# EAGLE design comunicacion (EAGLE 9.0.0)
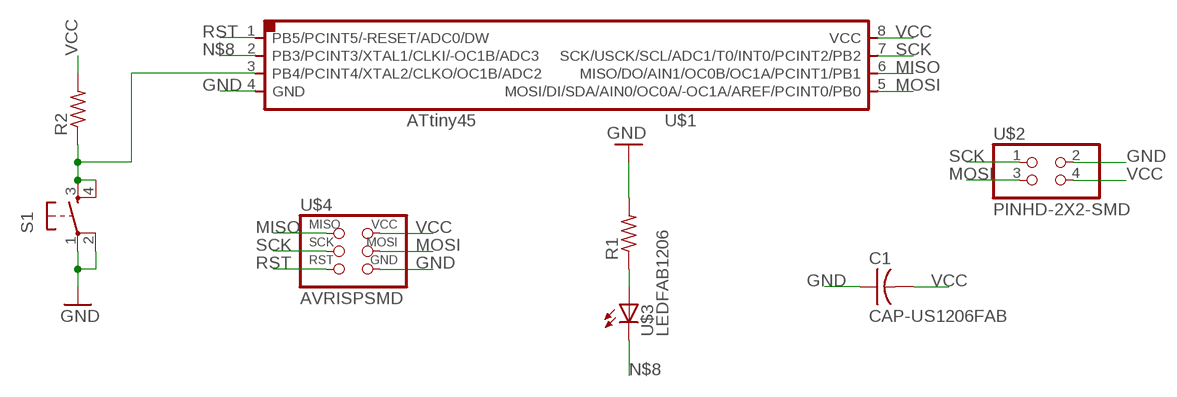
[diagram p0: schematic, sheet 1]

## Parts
C1  CAP-US1206FAB  [C1206FAB]
R1  RES-US1206FAB  [R1206FAB]
R2  RES-US1206FAB  [R1206FAB]
S1  6MM_SWITCH6MM_SWITCH  [6MM_SWITCH]
U$1  ATTINY45SI  [SOIC8]
U$2  PINHD-2X2-SMD  [2X02SMD]
U$3  LEDFAB1206  [LED1206FAB]
U$4  AVRISPSMD  [2X03SMD]

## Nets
GND: C1.1 R1.2 S1.1(P) S1.2(P1) U$1.4(GND) U$2.2 U$4.6(GND)
MISO: U$1.6(MISO/DO/AIN1/OC0B/OC1A/PCINT1/PB1) U$4.1(MISO)
MOSI: U$1.5(MOSI/DI/SDA/AIN0/OC0A/-OC1A/AREF/PCINT0/PB0) U$2.3 U$4.4(MOSI)
N$2: R2.1 S1.3(S) S1.4(S1) U$1.3(PB4/PCINT4/XTAL2/CLKO/OC1B/ADC2)
N$7: R1.1 U$3.1(A)
N$8: U$1.2(PB3/PCINT3/XTAL1/CLKI/-OC1B/ADC3) U$3.2(C)
RST: U$1.1(PB5/PCINT5/-RESET/ADC0/DW) U$4.5(RST)
SCK: U$1.7(SCK/USCK/SCL/ADC1/T0/INT0/PCINT2/PB2) U$2.1 U$4.3(SCK)
VCC: C1.2 R2.2 U$1.8(VCC) U$2.4 U$4.2(VCC)

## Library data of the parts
C1 = fab:CAP-US
R1 R2 = fab:RES-US: Resistor (US Symbol)
S1 = fab:6MM_SWITCH: OMRON SWITCH
U$1 = fab:ATTINY45
U$2 = fab:PINHD-2X2-SMD
U$3 = fab:LED: LED
U$4 = fab:AVRISP

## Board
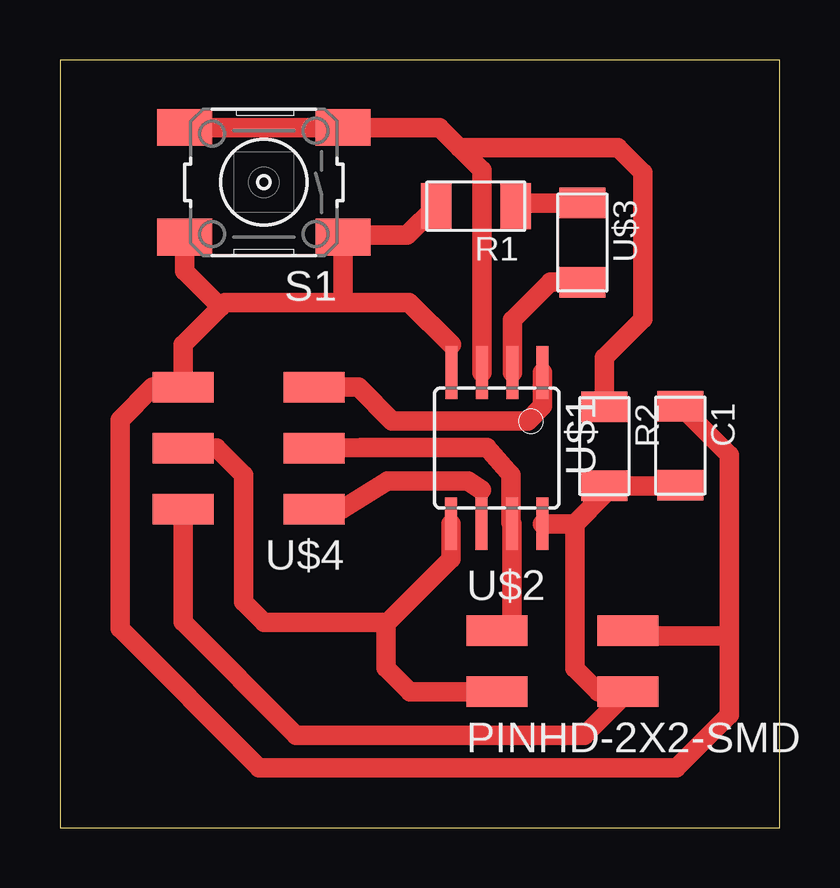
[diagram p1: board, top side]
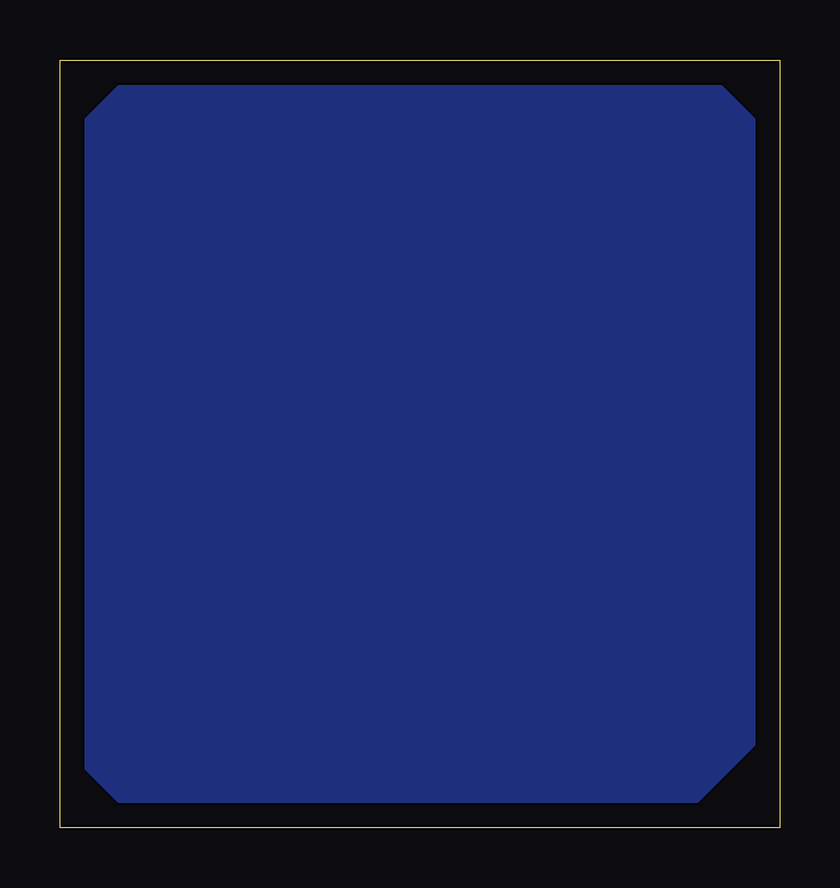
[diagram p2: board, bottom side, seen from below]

Size 30 x 32 mm. Coordinates in mm from the lower left corner, seen from the top.
Outline: 0,0 30,0 30,32 0,32 0,0
Copper layers (1*16): Top 0.035mm / dielectric 1.5mm / Bottom 0.035mm
Design rules "default": minimum track width 6mil, minimum drill 0.35mm, track to track 6mil, track to pad 6mil, pad to pad 6mil, via to via 6mil, smd to smd 6mil, copper to edge 40mil, drill to drill 6mil, minimum pad ring 10mil, minimum via ring 8mil, stop-mask expansion 4mil, vias tented up to drill 0mil, thermal gap 10mil

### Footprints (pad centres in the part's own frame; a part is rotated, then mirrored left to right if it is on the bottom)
C1206FAB = smd 1.27 x 1.905: 1 -1.651,0; 2 1.651,0
R1206FAB = smd 1.27 x 1.905: 1 -1.651,0; 2 1.651,0
6MM_SWITCH = smd 2.286 x 1.524: 1 -3.302,2.286; 2 3.302,2.286; 3 -3.302,-2.286; 4 3.302,-2.286
SOIC8 = smd 0.5 x 2.2: 1 -1.905,-3.154; 2 -0.645,-3.154; 3 0.625,-3.154; 4 1.895,-3.154; 5 1.905,3.154; 6 0.635,3.154; 7 -0.635,3.154; 8 -1.905,3.154
2X02SMD = smd 2.54 x 1.27: 1 -2.54,1.27; 2 2.92,1.27; 3 -2.54,-1.27; 4 2.92,-1.27
LED1206FAB = smd 1.27 x 1.905: 1 -1.651,0; 2 1.651,0
2X03SMD = smd 2.54 x 1.27: 1 -2.54,2.54; 2 2.92,2.54; 3 -2.54,0; 4 2.92,0; 5 -2.54,-2.54; 6 2.92,-2.54

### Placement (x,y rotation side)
C1  25.86,15.92 270 top
R1  17.34,25.91 180 top
R2  22.7,15.9 270 top
S1  8.5,26.9 180 top
U$1  18.21,15.82 180 top
U$2  20.75,6.93 0 top
U$3  21.78,24.39 270 top
U$4  8.05,15.82 180 top

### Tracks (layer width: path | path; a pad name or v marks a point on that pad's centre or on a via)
GND
  Top 0.508: U$1.4 16.32,20.14
  Top 0.813: 16.32,20.14 14.56,21.89 12,21.89 | R1.2 14.48,24.7 11.89,24.7 S1.1 11.8,22.09 12,21.89 | 12,21.89 6.89,21.89 6.7,21.7 | 6.7,21.7 5.13,20.13 U$4.6 3.86,18.36 2.5,17 2.5,8.3 8.3,2.5 25.7,2.5 27.9,4.7 27.9,8 | S1.2 5.2,23.2 6.7,21.7 | C1.1 27.9,15.53 27.9,8 | U$2.2 23.87,8 27.9,8
MISO
  Top 0.406: U$1.6 17.57,14.07
  Top 0.61: 11.78,13.28 U$4.1
  Top 0.813: 17.57,14.07 17,14.45 13.65,14.45 11.78,13.28
MOSI
  Top 0.508: U$4.4 6.53,15.82
  Top 0.61: 14.6,5.65 14.61,5.66 | 13.55,8.55 13.6,8.5
  Top 0.813: U$1.5 16.3,11.21 13.6,8.5 13.6,6.65 14.6,5.65 | 14.61,5.66 U$2.3 | 6.53,15.82 7.65,14.7 7.65,9.4 8.5,8.55 13.55,8.55
N$1
  pour Bottom: 6,31 27,31 29,29 29,3 27,1 4,1 1,4 1,29 3,31
N$2
  Top 0.813: U$1.3 17.59,27.41 16.65,28.35 | 16.65,28.35 15.81,29.19 S1.3 S1.4 | R2.1 22.7,19.6 24.3,21.2 24.3,27.3 23.25,28.35 16.65,28.35
N$7
  Top 0.813: U$3.1 19.12,26.04 R1.1
N$8
  Top 0.813: U$1.2 18.86,21.16 20.44,22.74 U$3.2
RST
  Top 0.813: U$4.5 12.44,18.36 13.85,16.95 19.5,16.95 20.11,17.57 U$1.1
SCK
  Top 0.61: 18.84,8.24 18.8,8.2 U$2.1 | 10.62,15.85 U$4.3 11.57,15.82 | 18.8,12.71 U$1.7
  Top 0.813: U$1.7 18.84,8.24 | 11.57,15.82 12.55,15.85 17.8,15.85 18.8,14.7 18.8,12.71
VCC
  Top 0.508: 22.44,5.66 U$2.4
  Top 0.813: U$1.8 21.47,12.67 | 21.47,12.67 21.47,6.63 22.44,5.66 | U$2.4 21.86,3.85 9.85,3.85 5.13,8.57 U$4.2 | 21.47,12.67 22.7,13.9 R2.2 25.84,14.25 C1.2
